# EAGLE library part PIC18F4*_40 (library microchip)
USB Microcontrollers with nanoWatt Technology High-Performance, Enhanced Flash, 28/40/44-Pin, Source: http://ww1.microchip.com/downloads/en/devicedoc/39632c.pdf
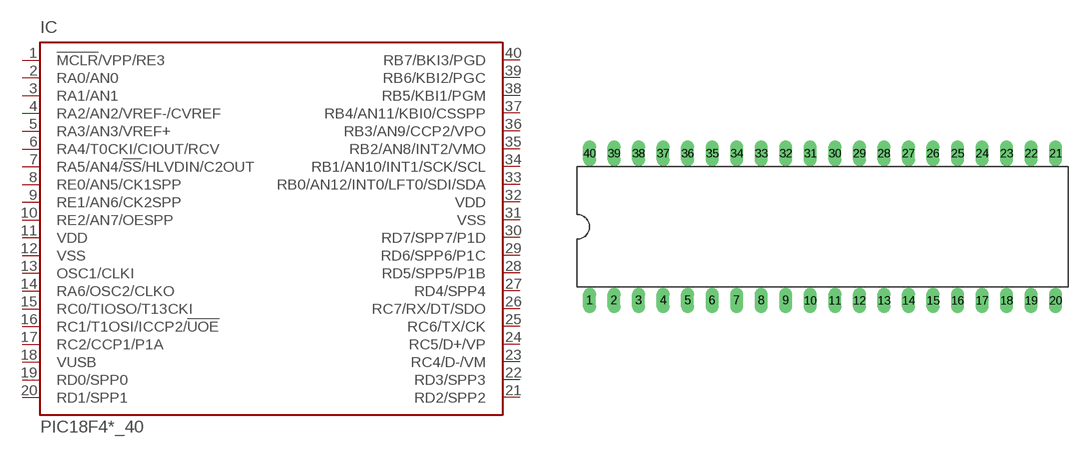
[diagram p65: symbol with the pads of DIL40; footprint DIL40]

Designator prefix IC

## PIC18F4455_40 (MF: MICROCHIP; MPN: PIC18F4455-I/P; OC_FARNELL: 9321314; OC_NEWARK: 05K2028), PIC18F4550_40 (MF: MICROCHIP; MPN: PIC18F4550-I/P; OC_FARNELL: 9321357; OC_NEWARK: 74K8623)  [DIL40]
1  !MCLR!/VPP/RE3  in
2  RA0/AN0
3  RA1/AN1
4  RA2/AN2/VREF-/CVREF
5  RA3/AN3/VREF+
6  RA4/T0CKI/CIOUT/RCV
7  RA5/AN4/!SS!/HLVDIN/C2OUT
8  RE0/AN5/CK1SPP
9  RE1/AN6/CK2SPP
10  RE2/AN7/OESPP
11  VDD  pwr
12  VSS  pwr
13  OSC1/CLKI  in
14  RA6/OSC2/CLKO  out
15  RC0/TIOSO/T13CKI
16  RC1/T1OSI/ICCP2/!UOE
17  RC2/CCP1/P1A
18  VUSB
19  RD0/SPP0
20  RD1/SPP1
21  RD2/SPP2
22  RD3/SPP3
23  RC4/D-/VM
24  RC5/D+/VP
25  RC6/TX/CK
26  RC7/RX/DT/SDO
27  RD4/SPP4
28  RD5/SPP5/P1B
29  RD6/SPP6/P1C
30  RD7/SPP7/P1D
31  VSS  pwr
32  VDD  pwr
33  RB0/AN12/INT0/LFT0/SDI/SDA
34  RB1/AN10/INT1/SCK/SCL
35  RB2/AN8/INT2/VMO
36  RB3/AN9/CCP2/VPO
37  RB4/AN11/KBI0/CSSPP
38  RB5/KBI1/PGM
39  RB6/KBI2/PGC
40  RB7/BKI3/PGD

## Footprint DIL40 (pad centres in mm)
Dual In Line package type P
drill 0.813 long: 1 -24.13,-7.62; 2 -21.59,-7.62; 3 -19.05,-7.62; 4 -16.51,-7.62; 5 -13.97,-7.62; 6 -11.43,-7.62; 7 -8.89,-7.62; 8 -6.35,-7.62; 9 -3.81,-7.62; 10 -1.27,-7.62; 11 1.27,-7.62; 12 3.81,-7.62; 13 6.35,-7.62; 14 8.89,-7.62; 15 11.43,-7.62; 16 13.97,-7.62; 17 16.51,-7.62; 18 19.05,-7.62; 19 21.59,-7.62; 20 24.13,-7.62; 21 24.13,7.62; 22 21.59,7.62; 23 19.05,7.62; 24 16.51,7.62; 25 13.97,7.62; 26 11.43,7.62; 27 8.89,7.62; 28 6.35,7.62; 29 3.81,7.62; 30 1.27,7.62; 31 -1.27,7.62; 32 -3.81,7.62; 33 -6.35,7.62; 34 -8.89,7.62; 35 -11.43,7.62; 36 -13.97,7.62; 37 -16.51,7.62; 38 -19.05,7.62; 39 -21.59,7.62; 40 -24.13,7.62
